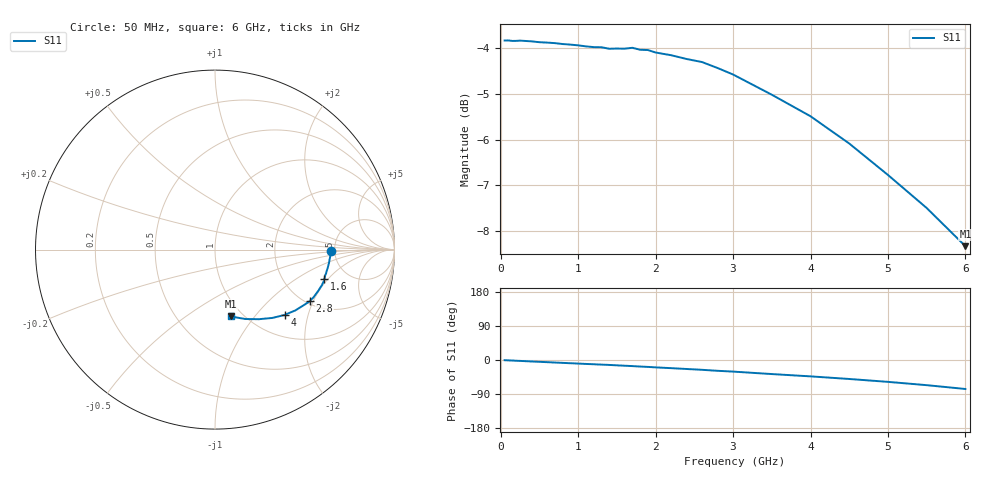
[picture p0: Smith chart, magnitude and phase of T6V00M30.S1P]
! SIEMENS Discrete & RF Semiconductors
! BAT62
! Si Schottky Diode in SOT143
! IF = 0.3 mA
! S-Parameters:  February  1997
# GHz  S  MA  R  50
!  f  S11
! GHz  MAG  ANG
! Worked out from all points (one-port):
!   34 points, 50 MHz to 6 GHz, reference 50 ohm
!   lowest |S11| = -8.3 dB at 6 GHz (marker M1), VSWR 2.24, Z = 44.1 - j38.5 ohm
!   |S11| at or under -10 dB: nowhere
!   S11 on the Smith chart (normalised r, x): 50 MHz: 4.61, -0.09; 1.6 GHz: 3.35, -1.83; 2.8 GHz: 2.10, -1.88; 4 GHz: 1.41, -1.43; 6 GHz: 0.88, -0.77
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0.05  0.6438 -0.5
0.15  0.643 -1.4
0.2  0.6431 -2.0
0.25  0.6436 -2.4
0.4  0.6424 -3.9
0.7  0.6395 -6.7
0.8  0.638 -7.6
1  0.6359 -9.4
1.1  0.6343 -10.4
1.2  0.6331 -11.2
1.3  0.6329 -12.2
1.4  0.6305 -13.0
1.6  0.6306 -15.1
1.7  0.632 -16.1
1.8  0.6289 -17.3
1.9  0.6285 -18.2
2  0.6245 -19.5
2.2  0.6203 -21.5
2.4  0.6144 -23.7
2.6  0.6097 -25.9
2.8  0.6006 -28.5
3  0.5909 -30.6
3.5  0.5615 -37.1
4  0.5318 -43.2
4.5  0.4965 -50.1
5  0.4587 -57.7
5.5  0.422 -66.4
6  0.3833 -76.5
